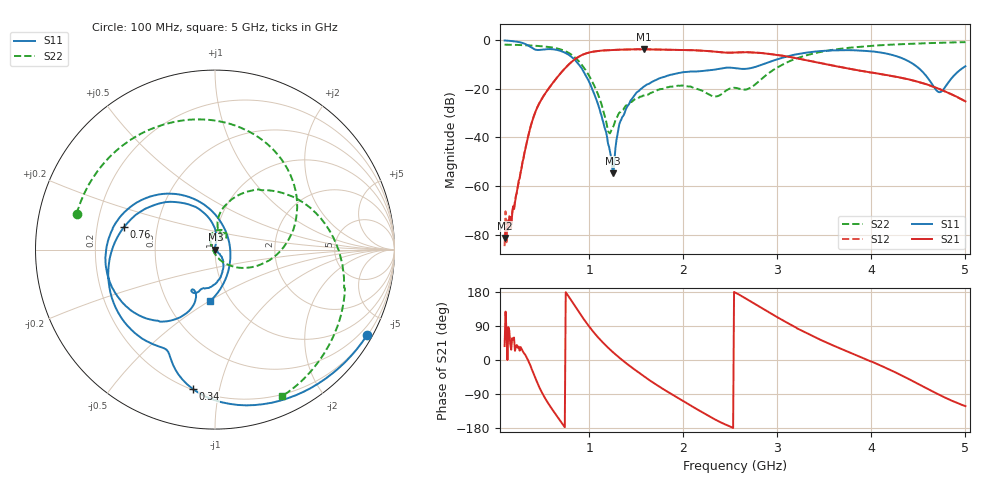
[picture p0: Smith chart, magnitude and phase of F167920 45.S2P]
!  2-Port S-parameters saved by WinCal
! VAR MeasName=S-Parameters (CALIBRATED_DATA) read from VNA (N5242A)
! VAR MeasDate=2016-11-22 9:57:44
! VAR NAME=F167920 45
! VAR FILENAME=F167920 45.S2P
! VAR DATE=2016-11-22 9:57:44
! VAR PHYS_PORTS=1,2
# Hz S DB R 50
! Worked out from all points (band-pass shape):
!   491 points, 100 MHz to 5 GHz, reference 50 ohm
!   highest |S21| = -3.86 dB at 1.58 GHz (marker M1); lowest = -81.3 dB at 100 MHz (marker M2)
!   |S21| within 3 dB of the highest: 891.7 MHz to 3.109 GHz (2.217 GHz wide, 111 % of centre)
!   lowest |S11| = -54.8 dB at 1.25 GHz (marker M3), VSWR 1.00, Z = 50.2 - j0.0176 ohm
!   |S11| at or under -10 dB: 886.8 MHz to 2.851 GHz (1.964 GHz wide, 105 % of centre); 4.448 GHz to end of sweep
!   |S22| runs from -38.4 to -0.9 dB; largest |S21 - S12| = 0.0023
!   S11 on the Smith chart (normalised r, x): 100 MHz: 0.22, -3.82; 340 MHz: 0.20, -0.83; 760 MHz: 0.32, +0.11; 5 GHz: 0.81, -0.50
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1e8  -0.25 -29.3  -81.30 36.7  -84.63 -154.8  -1.98 165.5
1.9e8  -0.55 -55.1  -68.24 54.3  -68.90 46.0  -2.04 152.3
3.4e8  -2.09 -99.0  -41.26 4.7  -41.24 4.1  -2.23 129.0
4.7e8  -4.15 -118.5  -25.93 -72.4  -25.92 -72.2  -2.55 106.8
6.4e8  -4.01 -157.6  -16.30 -142.3  -16.29 -142.3  -3.38 71.3
7.6e8  -5.63 166.1  -10.95 175.3  -10.95 175.2  -4.90 39.1
9.2e8  -11.69 114.2  -6.26 115.9  -6.25 115.9  -10.21 -11.2
1.09e9  -26.06 82.0  -4.59 60.9  -4.59 60.9  -22.06 -59.0
1.2e9  -42.63 97.4  -4.23 32.5  -4.23 32.5  -37.43 -121.2
1.25e9  -54.76 -5.5  -4.13 21.1  -4.13 21.1  -35.99 155.4
1.34e9  -32.75 -43.8  -4.01 1.9  -4.01 2.0  -29.15 126.7
1.58e9  -19.19 -65.0  -3.86 -42.8  -3.86 -42.8  -22.86 107.2
1.74e9  -15.90 -79.8  -3.96 -69.3  -3.95 -69.3  -20.41 96.2
2.18e9  -12.86 -108.0  -4.40 -134.9  -4.40 -134.9  -20.57 47.7
2.55e9  -11.60 -120.0  -5.20 178.3  -5.19 178.3  -19.69 62.3
2.95e9  -8.62 -112.9  -5.94 120.0  -5.92 119.9  -12.53 79.0
3.37e9  -4.94 -140.7  -8.84 63.7  -8.80 63.5  -5.72 35.4
3.8e9  -4.25 -174.9  -12.11 16.6  -12.09 16.3  -3.10 -3.0
4.19e9  -5.88 148.8  -14.62 -25.0  -14.67 -25.3  -2.01 -28.2
4.47e9  -10.59 110.8  -16.92 -59.5  -16.94 -59.7  -1.54 -42.9
4.72e9  -21.46 10.6  -20.10 -91.5  -20.13 -91.4  -1.21 -54.2
5e9  -10.84 -95.3  -25.22 -121.7  -25.23 -121.7  -0.94 -65.5
